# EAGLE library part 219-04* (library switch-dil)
Surface Mount DIP Switch Series 219 SMT CTS Electronic Components Sourc: www.ctscorp.com
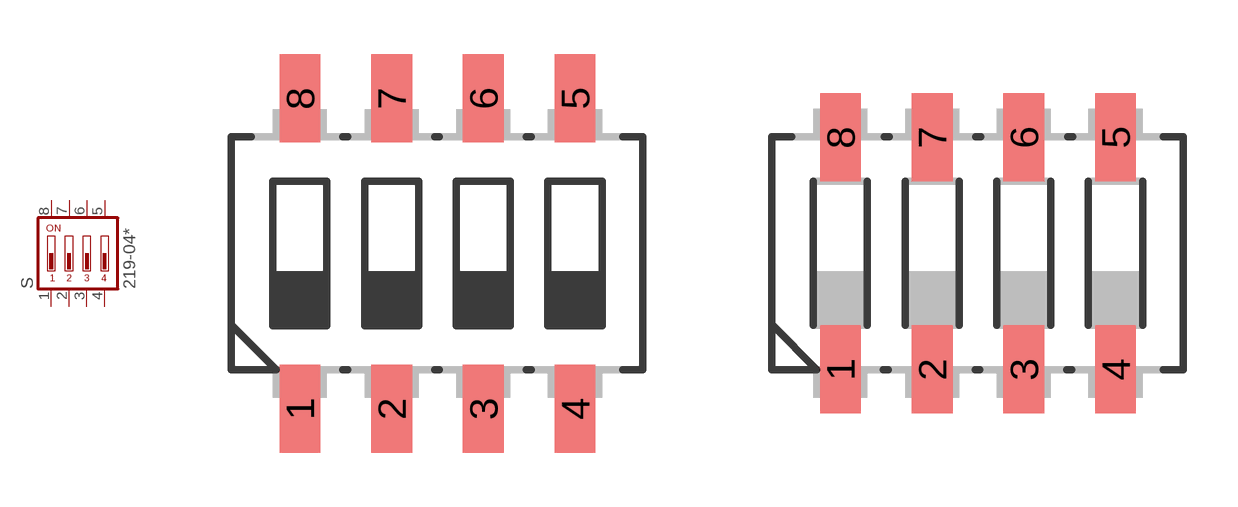
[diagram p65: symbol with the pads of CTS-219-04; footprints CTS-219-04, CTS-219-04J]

Designator prefix S

## 219-04 (OC_FARNELL: unknown; OC_NEWARK: unknown)  [CTS-219-04]
1  1  pas
2  2  pas
3  3  pas
4  4  pas
5  5  pas
6  6  pas
7  7  pas
8  8  pas

## 219-04J (OC_FARNELL: unknown; OC_NEWARK: unknown)  [CTS-219-04J]
Pads as for CTS-219-04

## Footprint CTS-219-04 (pad centres in mm)
Surface Mount DIP Switch Series 219 SMT CTS Electronic Components Sourc: www.ctscorp.com
smd 1.13 x 2.44: 1 -3.81,-4.3; 2 -1.27,-4.3; 3 1.27,-4.3; 4 3.81,-4.3; 5 3.81,4.3; 6 1.27,4.3; 7 -1.27,4.3; 8 -3.81,4.3

## Footprint CTS-219-04J (pad centres in mm)
Surface Mount DIP Switch Series 219 SMT "J" Bend CTS Electronic Components Sourc: www.ctscorp.com
smd 1.13 x 2.44: 1 -3.81,-3.215; 2 -1.27,-3.215; 3 1.27,-3.215; 4 3.81,-3.215; 5 3.81,3.215; 6 1.27,3.215; 7 -1.27,3.215; 8 -3.81,3.215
